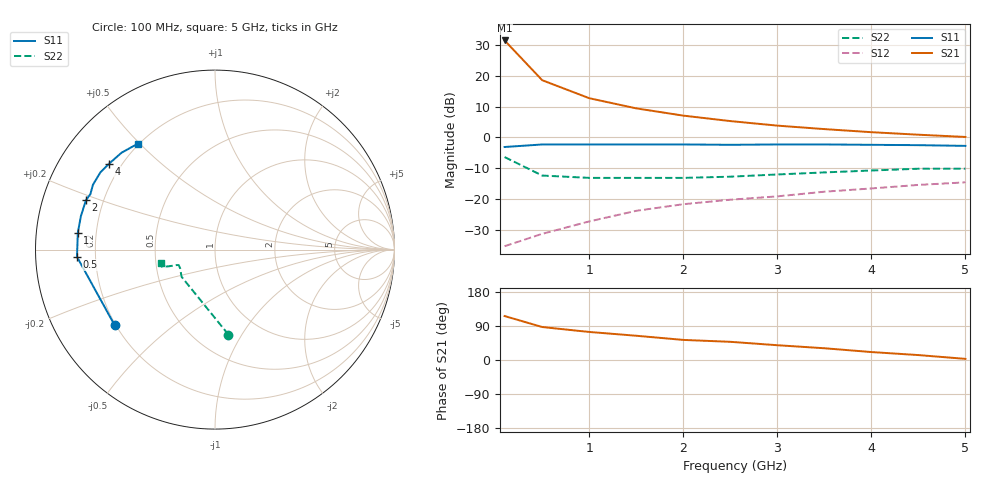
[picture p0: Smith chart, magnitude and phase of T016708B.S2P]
!AT-01670
!S-PARAMETERS at Vce=8V  Ic=60mA.  LAST UPDATED 07-21-92
!OBSOLETED Feb 1994 - nearest replacement: AT-42070
# ghz s ma r 50
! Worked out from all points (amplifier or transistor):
!   11 points, 100 MHz to 5 GHz, reference 50 ohm
!   highest |S21| = 31.6 dB at 100 MHz (marker M1)
!   |S21| within 3 dB of that: start of sweep to 192.7 MHz
!   unconditionally stable (mu >= 1): 582.2 MHz to end of sweep
!   at 500 MHz: K = 0.96, MSG = 25.0 dB, |S12| = -31.4 dB
!   at 2.5 GHz: K = 1.27, MAG = 9.7 dB, |S12| = -20.3 dB
!   at 5 GHz: K = 1.18, MAG = 4.8 dB, |S12| = -14.6 dB
!   S11 on the Smith chart (normalised r, x): 100 MHz: 0.20, -0.32; 500 MHz: 0.13, -0.03; 1 GHz: 0.13, +0.06; 2 GHz: 0.13, +0.18; 4 GHz: 0.15, +0.35; 5 GHz: 0.20, +0.49
0.1  0.7 -143.0  38.01 116.0  0.017 40.0  0.48 -81.0
0.5  0.77 -177.0  8.56 87.0  0.027 49.0  0.24 -141.0
1  0.77 173.0  4.36 74.0  0.043 59.0  0.22 -152.0
1.5  0.77 166.0  2.98 64.0  0.064 58.0  0.22 -155.0
2  0.77 159.0  2.27 53.0  0.082 59.0  0.22 -157.0
2.5  0.76 156.0  1.85 48.0  0.097 61.0  0.23 -158.0
3  0.77 152.0  1.56 39.0  0.11 57.0  0.25 -159.0
3.5  0.77 146.0  1.37 31.0  0.131 54.0  0.27 -160.0
4  0.76 141.0  1.22 21.0  0.148 51.0  0.29 -161.0
4.5  0.75 134.0  1.11 13.0  0.169 45.0  0.31 -162.0
5  0.73 126.0  1.02 3.0  0.186 41.0  0.31 -166.0
